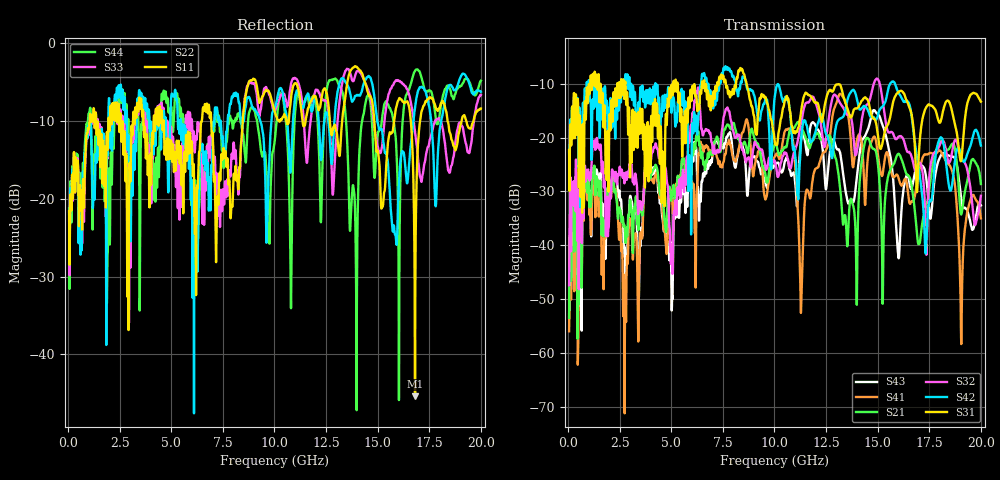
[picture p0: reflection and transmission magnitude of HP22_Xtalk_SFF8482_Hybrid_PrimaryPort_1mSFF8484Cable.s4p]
# MHz S MA R 50.00
! FREQ  S11  S12  S13  S14
!  S21  S22  S23  S24
!  S31  S32  S33  S34
!  S41  S42  S43  S44
!  MAG  ANG  MAG  ANG  MAG  ANG  MAG  ANG
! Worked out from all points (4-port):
!   1996 points, 50 MHz to 20 GHz, reference 50 ohm
!   strongest paths, dB at 50 MHz, 5.04 GHz, 10.03 GHz, 15.02 GHz, 20 GHz:
!     S31: -22.3, -10.8, -21.3, -19.8, -13.3
!     S42: -22.6, -13.6, -12.0, -15.7, -21.5
!     S32: -47.4, -43.4, -24.6, -9.2, -30.8
!     S21: -53.4, -30.6, -21.3, -25.3, -28.6
!     S41: -56.0, -30.4, -23.5, -23.5, -35.0
!     S43: -53.6, -49.5, -25.1, -15.6, -32.6
!   lowest |S11| = -45.4 dB at 16.81 GHz (marker M1), VSWR 1.01, Z = 49.9 + j0.517 ohm
!   |S11| at or under -10 dB: start of sweep to 1.041 GHz; 4.624 GHz to 6.482 GHz (1.858 GHz wide, 33.5 % of centre); 6.934 GHz to 8.459 GHz (1.525 GHz wide, 19.8 % of centre)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
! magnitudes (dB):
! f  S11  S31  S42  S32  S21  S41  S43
! 50 MHz  -21.6  -22.3  -22.6  -47.4  -53.4  -56.0  -53.6
! 3.85 GHz  -15.7  -17.2  -12.0  -22.5  -23.5  -23.2  -22.8
! 5.01 GHz  -13.3  -10.3  -15.4  -42.0  -31.2  -29.7  -49.3
! 6.26 GHz  -18.3  -15.0  -19.2  -11.7  -20.5  -28.7  -29.0
! 13.93 GHz  -3.0  -14.6  -11.9  -23.3  -38.0  -21.9  -29.5
! 16.81 GHz  -45.4  -22.2  -21.2  -26.1  -34.0  -30.7  -26.4
! 20 GHz  -8.4  -13.3  -21.5  -30.8  -28.6  -35.0  -32.6
